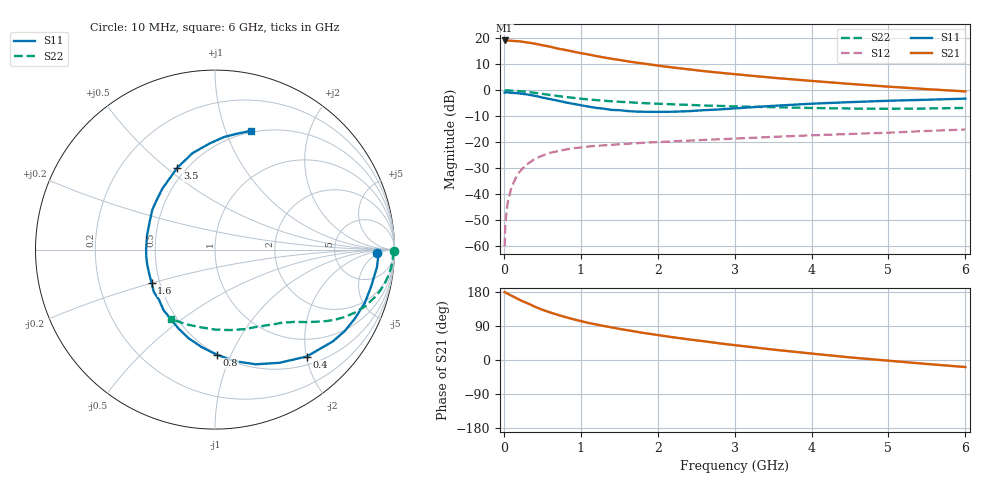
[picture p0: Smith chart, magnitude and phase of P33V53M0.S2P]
! SIEMENS Small Signal Semiconductors
! BFP181
! Si NPN RF Bipolar Junction Transistor in SOT143
! VCE = 3.5 V  IC = 3 mA
! Common Emitter S-Parameters:  March  1996
# GHz  S  MA  R  50
!  f  S11  S21  S12  S22
! GHz  MAG  ANG  MAG  ANG  MAG  ANG  MAG  ANG
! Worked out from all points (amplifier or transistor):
!   36 points, 10 MHz to 6 GHz, reference 50 ohm
!   highest |S21| = 19.2 dB at 10 MHz (marker M1)
!   |S21| within 3 dB of that: start of sweep to 683.7 MHz
!   unconditionally stable (mu >= 1): 2.127 GHz to end of sweep
!   at 250 MHz: K = 0.15, MSG = 24.3 dB, |S12| = -30.0 dB
!   at 1.4 GHz: K = 0.76, MSG = 16.6 dB, |S12| = -21.0 dB
!   at 6 GHz: K = 1.09, MAG = 5.5 dB, |S12| = -15.1 dB
!   lowest NFmin = 1.40 dB at 450 MHz
!   S11 on the Smith chart (normalised r, x): 10 MHz: 19, -4; 400 MHz: 0.65, -2.00; 800 MHz: 0.50, -0.89; 1.6 GHz: 0.45, -0.20; 3.5 GHz: 0.45, +0.54; 6 GHz: 0.48, +1.22
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0.01  0.9049 -1.3  9.098 179.0  0.001 93.5  0.9946 -0.5
0.02  0.9103 -2.8  9.042 178.3  0.0028 80.8  0.9929 -1.1
0.05  0.9073 -6.3  9.053 174.7  0.0069 89.8  0.9919 -2.9
0.1  0.8941 -13.2  8.954 169.7  0.0137 82.4  0.9868 -5.8
0.2  0.8695 -26.0  8.781 159.4  0.0265 74.7  0.9642 -11.3
0.25  0.8535 -32.1  8.566 154.5  0.0318 72.0  0.9488 -13.9
0.4  0.7847 -49.4  7.904 140.9  0.0474 62.2  0.8944 -20.7
0.5  0.7255 -60.4  7.381 132.7  0.0554 56.8  0.8529 -24.4
0.6  0.6779 -70.5  6.916 125.6  0.0624 52.8  0.8126 -27.6
0.7  0.6321 -79.8  6.352 119.3  0.0674 48.8  0.7765 -30.1
0.8  0.5865 -88.8  5.964 113.2  0.0722 46.0  0.7448 -32.2
1  0.5164 -106.3  5.184 102.7  0.0793 40.8  0.6893 -35.7
1.1  0.485 -114.7  4.886 97.9  0.0828 38.8  0.6664 -37.2
1.3  0.443 -130.3  4.288 89.8  0.087 35.8  0.6298 -39.8
1.6  0.3991 -152.2  3.628 78.9  0.0935 32.7  0.5903 -43.1
1.8  0.3869 -167.3  3.291 71.9  0.0972 31.4  0.5688 -45.4
2.2  0.3867 168.4  2.738 60.0  0.1043 29.1  0.5372 -50.3
2.8  0.428 138.8  2.182 44.0  0.1141 26.7  0.5006 -58.5
3.5  0.5019 114.8  1.741 27.5  0.1269 24.0  0.4727 -69.7
4.5  0.5916 93.0  1.326 6.9  0.1442 19.4  0.4457 -89.6
5.5  0.6577 79.2  1.052 -10.5  0.1648 15.6  0.4461 -111.1
6  0.6905 73.3  0.951 -18.6  0.1759 12.8  0.4573 -122.2
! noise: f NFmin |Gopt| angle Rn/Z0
0.45  1.4  0.56  17  0.36
0.9  1.5  0.45  35  0.34
1.8  1.85  0.25  82  0.36
